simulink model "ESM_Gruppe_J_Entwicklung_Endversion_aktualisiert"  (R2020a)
settings: Solver=VariableStepAuto  StartTime=0  StopTime=Simulation  RelTol=1e-3
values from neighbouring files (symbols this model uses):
  c = [0;0]    [Testskript_Manoeverauswahl.m]
  ch = 100000    [Single_TestSkript_Hinterachse.m]    (also in Testskript_Hinterachse.m = 0)
  cv = 80000    [Single_Testskript_Vorderachse.m]    (also in Testskript_Vorderachse.m = (b-a).*rand(1,1) + a)
  Jzz = 1    [Single_Testskript_Karosserie.m]    (also in Testskript_Karosserie.m = (b-a).*rand(1,1) + a)
  lh = 1.3    [Single_TestSkript_Hinterachse.m]    (also in Testskript_Hinterachse.m = (b-a).*rand(1,1) + a; Single_Testskript_Karosserie.m; Testskript_Karosserie.m = (b-a).*rand(1,1) + a)
  lv = 1.3    [Single_Testskript_Karosserie.m]    (also in Testskript_Karosserie.m = (b-a).*rand(1,1) + a; Single_Testskript_Vorderachse.m = 1.5; Testskript_Vorderachse.m = (b-a).*rand(1,1) + a)
  m = 1500    [Single_Testskript_Karosserie.m]    (also in Testskript_Karosserie.m = (b-a).*rand(1,1) + a)

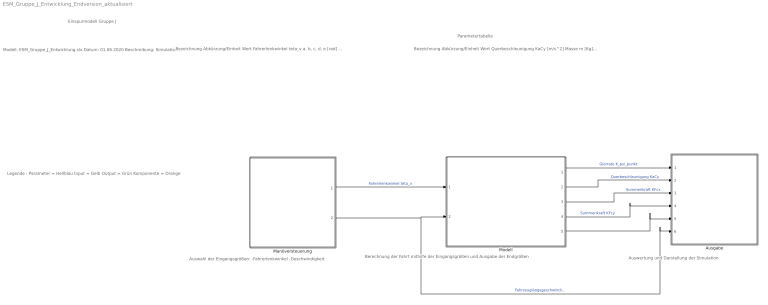
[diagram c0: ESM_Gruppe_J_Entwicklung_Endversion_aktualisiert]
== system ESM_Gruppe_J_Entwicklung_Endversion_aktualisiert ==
  note: Modell: ESM_Gruppe_J_Entwicklung.slx Datum: 01.06.2020 Beschreibung: Simulation der linearen Fahrdynamik Implementierung: Simulink 2019b (2019a) Autor: Alexander Gossen, Hermine Makou Bemerkung: Prototyp Letzte Änderung: 01.06.2020
  note: Bezeichnung Abkürzung/Einheit Wert Fahrerlenkwinkel teta_v a, b, c, d, e [rad] Fahrerlenkwinkel (hinten) teta_h 0 Fahrzeuglängsgeschwindigkeit KvCx a, b, c, d, e [m/s] Schwimmwinkel (vorne/hinten) beta, beta_v, beta_h [rad] Achschräglaufwinkel (vorne/hinten) Alpha_v, Alpha_h [rad] Seitenführungskraft (vorne/hinten) RFyv, RFyh [F] Gierrate K_psi_punkt
  note: Parametertabelle
  note: Einspurmodell Gruppe J
  note: Auswertung und Darstellung der Simulation
  note: Berechnung der Fahrt mithilfe der Eingangsgrößen und Ausgabe der Endgrößen
  note: Auswahl der Eingangsgrößen: -Fahrerlenkwinkel -Geschwindigkeit
  note: Legende : Parameter = Hellblau Input = Gelb Output = Grün Komponente = Orange
  note: Bezeichnung Abkürzung/Einheit Wert Querbeschleunigung KaCy [m/s^2] Masse m [Kg] 1550 Massenträgheit Jzz [Kg/m^2] 2800 Achsensteifigkeit (vorne/hinten) cv, ch [N/rad] 75.000 (vorne), 150.000 (hinten) Schwerpunktabstand (vorne/hinten) lv, lh [m] 1.3 (vorne), 2.6 (hinten) Radstand l
  Ausgabe : Subsystem
  Manöversteuerung : Subsystem
  Modell : Subsystem
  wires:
  Manöversteuerung/1(Fahrerlenkwinkel teta_v) -> Modell/1(Fahrerlenkwinkel teta_v)  "Fahrerlenkwinkel teta_v"
  Manöversteuerung/2(Fahrzeuglängsgeschwindigkeit KvCx) -> Modell/2(Fahrzeuglängsgeschwindigkeit KvCx), Ausgabe/6(Schwimmwinkel beta)  "Fahrzeuglängsgeschwindigkeit KvCx"
  Modell/1(Gierrate K_psi_punkt) -> Ausgabe/1(Gierrate K_psi_punkt)  "Gierrate K_psi_punkt"
  Modell/2(Querbeschleunigung KaCy) -> Ausgabe/2(Querbeschleunigung KaCy)  "Querbeschleunigung KaCy"
  Modell/3(Summenkraft KFcx) -> Ausgabe/3(Summenkraft KFcx)  "Summenkraft KFcx"
  Modell/4(Summenkraft KFcy) -> Ausgabe/4(Summenkraft KFcy)  "Summenkraft KFcy"
  Modell/5(Schwimmwinkel beta) -> Ausgabe/5(Fahrzeuglängsgeschwindigkeit KvCx)

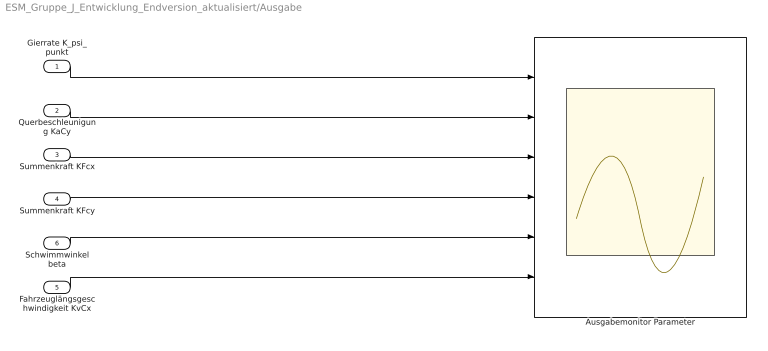
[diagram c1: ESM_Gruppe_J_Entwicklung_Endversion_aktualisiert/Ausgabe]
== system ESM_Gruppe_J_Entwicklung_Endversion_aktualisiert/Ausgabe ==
  Gierrate K_psi_punkt : Inport
  Querbeschleunigung KaCy : Inport  Port=2
  Summenkraft KFcx : Inport  Port=3
  Summenkraft KFcy : Inport  Port=4
  Fahrzeuglängsgeschwindigkeit KvCx : Inport  Port=5
  Schwimmwinkel beta : Inport  Port=6
  Ausgabemonitor Parameter : Scope  NumInputPorts=6
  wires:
  Gierrate K_psi_punkt/1 -> Ausgabemonitor Parameter/1
  Querbeschleunigung KaCy/1 -> Ausgabemonitor Parameter/2
  Summenkraft KFcx/1 -> Ausgabemonitor Parameter/3
  Summenkraft KFcy/1 -> Ausgabemonitor Parameter/4
  Schwimmwinkel beta/1 -> Ausgabemonitor Parameter/5
  Fahrzeuglängsgeschwindigkeit KvCx/1 -> Ausgabemonitor Parameter/6

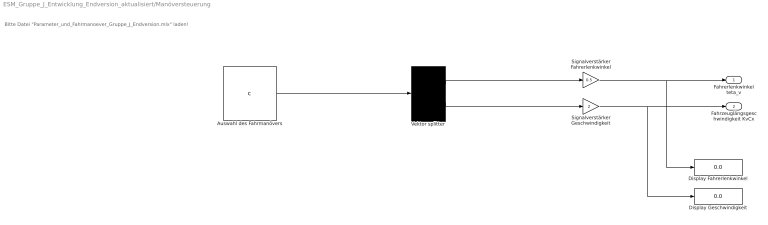
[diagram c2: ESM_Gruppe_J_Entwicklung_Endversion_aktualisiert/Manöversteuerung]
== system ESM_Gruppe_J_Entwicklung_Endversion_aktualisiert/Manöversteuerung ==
  note: Bitte Datei "Parameter_und_Fahrmanoever_Gruppe_J_Endversion.mlx" laden!
  Auswahl des Fahrmanövers : Constant  Value=c
  Display Fahrerlenkwinkel : Display
  Display Geschwindigkeit : Display
  Signalverstärker Fahrerlenkwinkel : Gain  Gain=0.5
  Signalverstärker Geschwindigkeit : Gain  Gain=2
  Vektor splitter : Demux  Outputs=2
  Fahrerlenkwinkel teta_v : Outport
  Fahrzeuglängsgeschwindigkeit KvCx : Outport  Port=2
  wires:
  Vektor splitter/1 -> Signalverstärker Fahrerlenkwinkel/1
  Vektor splitter/2 -> Signalverstärker Geschwindigkeit/1
  Signalverstärker Geschwindigkeit/1 -> Fahrzeuglängsgeschwindigkeit KvCx/1, Display Geschwindigkeit/1
  Signalverstärker Fahrerlenkwinkel/1 -> Fahrerlenkwinkel teta_v/1, Display Fahrerlenkwinkel/1
  Auswahl des Fahrmanövers/1 -> Vektor splitter/1

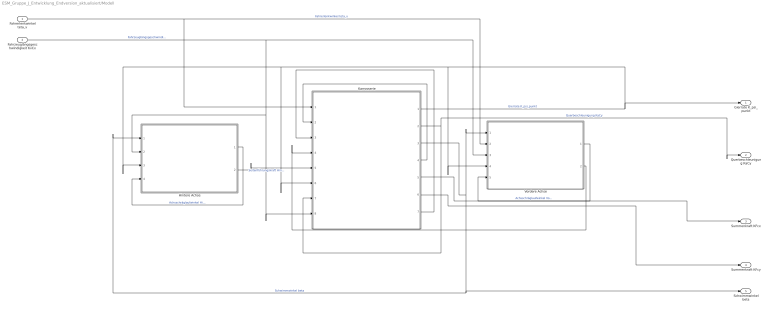
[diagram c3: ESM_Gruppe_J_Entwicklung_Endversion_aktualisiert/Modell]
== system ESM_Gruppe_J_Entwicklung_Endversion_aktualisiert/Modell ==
  Fahrerlenkwinkel teta_v : Inport
  Fahrzeuglängsgeschwindigkeit KvCx : Inport  Port=2
  Hintere Achse : Subsystem
  Karrosserie : Subsystem
  Vordere Achse : Subsystem
  Gierrate K_psi_punkt : Outport
  Querbeschleunigung KaCy : Outport  Port=2
  Summenkraft KFcx : Outport  Port=3
  Summenkraft KFcy : Outport  Port=4
  Schwimmwinkel beta : Outport  Port=5
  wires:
  Fahrerlenkwinkel teta_v/1 -> Vordere Achse/2(Fahrerlenkwinkel teta_v), Karrosserie/1(Fahrerlenkwinkel teta_v)  "Fahrerlenkwinkel teta_v"
  Fahrzeuglängsgeschwindigkeit KvCx/1 -> Vordere Achse/3(Geschwindigkeit KvCx), Karrosserie/8(Fahrzeuglängsgeschwindigkeit KvCx), Hintere Achse/2(Geschwindigkeit KvCx)  "Fahrzeuglängsgeschwindigkeit KvCx"
  Vordere Achse/1(Achsschräglaufwinkel vorderachse Alpha_v) -> Vordere Achse/5(Achsschräglaufwinkel vornerachse Alpha_v)  "Achsschräglaufwinkel Vorderachse Alpha_v"
  Hintere Achse/1(Achsschräglaufwinkel hinterachse alpha_v) -> Hintere Achse/4(Achsschräglaufwinkel hinterachse Alpha_h)  "Achsschräglaufwinkel Hinterachse Alpha_h"
  Vordere Achse/2(Seitenführungskraft vorderachse RFyv) -> Karrosserie/4(Seitenführungskraft vorderachse RFyv)
  Karrosserie/2(Querbeschleunigung kAcY) -> Karrosserie/7(Querbeschleunigung KaCy), Querbeschleunigung KaCy/1  "Querbeschleunigung KaCy"
  Karrosserie/1(Gierrate k_psi_punkt) -> Karrosserie/6(Gierrate K_psi_punkt), Hintere Achse/3(Gierrate K_psi_punkt), Vordere Achse/4(Gierrate K_psi_punkt), Gierrate K_psi_punkt/1  "Gierrate K_psi_punkt"
  Hintere Achse/2(Seitenführungskraft hinterachse RFyh) -> Karrosserie/5(Seitenführungskraft hintererachse RFyh)  "Seitenführungskraft Hinterachse RFyv"
  Karrosserie/6(Summenkraft KFcy) -> Summenkraft KFcy/1
  Karrosserie/5(Summenkraft KFcx) -> Summenkraft KFcx/1
  Karrosserie/4(Seitenführungskraft vorderachse KFyv) -> Karrosserie/2(Seitenführungskraft Vorderachse KFyv)
  Karrosserie/7(Seitenführungskraft hinterachse KFyh) -> Karrosserie/3(Seitenführungskraft Hinterachse KFyh)
  Karrosserie/3(Schwimmwinkel beta) -> Vordere Achse/1(Schwimmwinkel beta), Hintere Achse/1(Schwimmwinkel beta), Schwimmwinkel beta/1  "Schwimmwinkel beta"

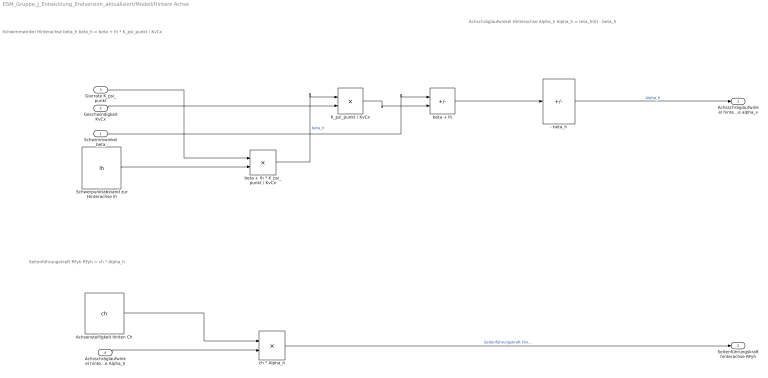
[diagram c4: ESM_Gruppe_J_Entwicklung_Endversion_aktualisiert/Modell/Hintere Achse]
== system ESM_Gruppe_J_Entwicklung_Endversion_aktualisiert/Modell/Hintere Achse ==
  note: Seitenführungskraft RFyh RFyh = ch * Alpha_h
  note: Schwimmwinkel Hinterachse beta_h beta_h = beta + Ih * K_psi_punkt / KvCx
  note: Achschräglaufwinkel Hinterachse Alpha_h Alpha_h = teta_h(0) - beta_h
  Schwimmwinkel beta : Inport
  Geschwindigkeit KvCx : Inport  Port=2
  Gierrate K_psi_punkt : Inport  Port=3
  Achsschräglaufwinkel hinterachse Alpha_h : Inport  Port=4
  - beta_h : Sum  Inputs=-
  Achsensteifigkeit hinten Ch : Constant  Value=ch
  K_psi_punkt / KvCx : Product  Inputs=*/
  Schwerpunktabstand zur Hinterachse lh : Constant  Value=lh
  beta + Ih : Sum  Inputs=+-
  beta + Ih * K_psi_punkt / KvCx : Product  Inputs=**
  ch * Alpha_h : Product
  Achsschräglaufwinkel hinterachse alpha_v : Outport
  Seitenführungskraft hinterachse RFyh : Outport  Port=2
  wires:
  - beta_h/1 -> Achsschräglaufwinkel hinterachse alpha_v/1  "Alpha_h"
  ch * Alpha_h/1 -> Seitenführungskraft hinterachse RFyh/1  "Seitenführungskraft Hinterachse RFyv"
  Achsensteifigkeit hinten Ch/1 -> ch * Alpha_h/1
  Achsschräglaufwinkel hinterachse Alpha_h/1 -> ch * Alpha_h/2
  beta + Ih * K_psi_punkt / KvCx/1 -> K_psi_punkt / KvCx/1  "beta_h"
  Geschwindigkeit KvCx/1 -> K_psi_punkt / KvCx/2
  beta + Ih/1 -> - beta_h/1
  Schwimmwinkel beta/1 -> beta + Ih/1
  K_psi_punkt / KvCx/1 -> beta + Ih/2
  Schwerpunktabstand zur Hinterachse lh/1 -> beta + Ih * K_psi_punkt / KvCx/2
  Gierrate K_psi_punkt/1 -> beta + Ih * K_psi_punkt / KvCx/1

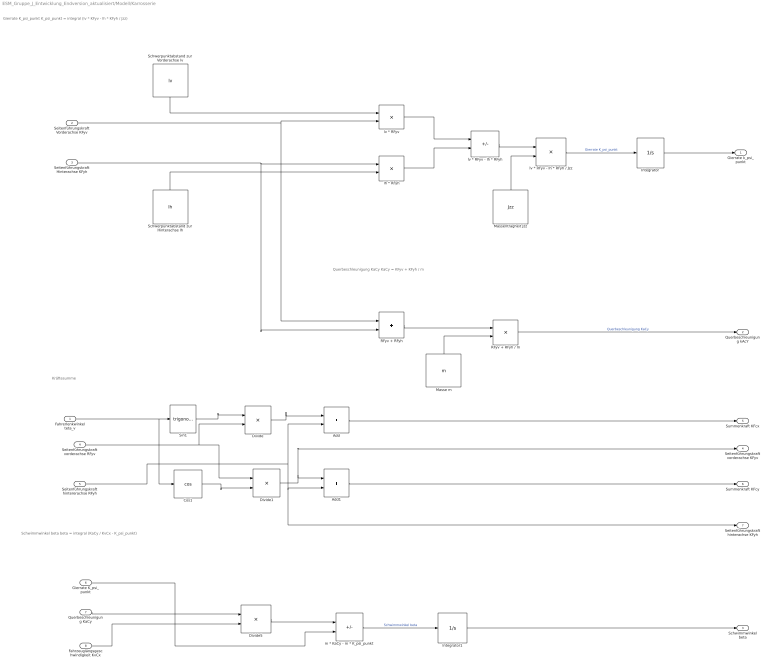
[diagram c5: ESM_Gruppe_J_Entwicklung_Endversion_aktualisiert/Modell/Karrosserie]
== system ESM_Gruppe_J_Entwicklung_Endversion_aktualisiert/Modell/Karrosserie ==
  note: Kräftesumme
  note: Gierrate K_psi_punkt K_psi_punkt = integral (lv * KFyv - lh * KFyh / Jzz)
  note: Querbeschleunigung KaCy KaCy = KFyv + KFyh / m
  note: Schwimmwinkel beta beta = integral (KaCy / KvCx - K_psi_punkt)
  Fahrerlenkwinkel teta_v : Inport
  Seitenführungskraft Vorderachse KFyv : Inport  Port=2
  Seitenführungskraft Hinterachse KFyh : Inport  Port=3
  Seitenführungskraft vorderachse RFyv : Inport  Port=4
  Seitenführungskraft hintererachse RFyh : Inport  Port=5
  Gierrate K_psi_punkt : Inport  Port=6
  Querbeschleunigung KaCy : Inport  Port=7
  Fahrzeuglängsgeschwindigkeit KvCx : Inport  Port=8
  Add : Sum
  Add1 : Sum
  Cos1 : Trigonometry  Operator=cos
  Divide : Product
  Divide1 : Product
  Divide5 : Product  Inputs=*/
  Integrator : Integrator
  Integrator1 : Integrator
  Masse m : Constant  Value=m
  Massenträgheit Jzz : Constant  Value=Jzz
  RFyv + RFyh : Sum
  RFyv + RFyh / m : Product  Inputs=*/
  Schwerpunktabstand zur Hinterachse lh : Constant  Value=lh
  Schwerpunktabstand zur Vorderachse lv : Constant  Value=lv
  Sin1 : Trigonometry
  lh * RFyh : Product
  lv * RFyv : Product
  lv * RFyv - lh * RFyh : Sum  Inputs=+-
  lv * RFyv - lh * RFyh / Jzz : Product  Inputs=*/
  m * KaCy - m * K_psi_punkt : Sum  Inputs=+-
  Gierrate k_psi_punkt : Outport
  Querbeschleunigung kAcY : Outport  Port=2
  Schwimmwinkel beta : Outport  Port=3
  Seitenführungskraft vorderachse KFyv : Outport  Port=4
  Summenkraft KFcx : Outport  Port=5
  Summenkraft KFcy : Outport  Port=6
  Seitenführungskraft hinterachse KFyh : Outport  Port=7
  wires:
  RFyv + RFyh / m/1 -> Querbeschleunigung kAcY/1  "Querbeschleunigung KaCy"
  m * KaCy - m * K_psi_punkt/1 -> Integrator1/1  "Schwimmwinkel beta"
  lv * RFyv - lh * RFyh/1 -> lv * RFyv - lh * RFyh / Jzz/1
  lv * RFyv/1 -> lv * RFyv - lh * RFyh/1
  Massenträgheit Jzz/1 -> lv * RFyv - lh * RFyh / Jzz/2
  lh * RFyh/1 -> lv * RFyv - lh * RFyh/2
  Schwerpunktabstand zur Vorderachse lv/1 -> lv * RFyv/1
  Schwerpunktabstand zur Hinterachse lh/1 -> lh * RFyh/2
  Masse m/1 -> RFyv + RFyh / m/2
  RFyv + RFyh/1 -> RFyv + RFyh / m/1
  Fahrerlenkwinkel teta_v/1 -> Cos1/1, Sin1/1
  Sin1/1 -> Divide/1
  Seitenführungskraft vorderachse RFyv/1 -> Divide1/1, Divide/2
  Divide/1 -> Add/1
  Seitenführungskraft hintererachse RFyh/1 -> Add/2, Seitenführungskraft hinterachse KFyh/1, Add1/2
  Add/1 -> Summenkraft KFcx/1
  Divide1/1 -> Seitenführungskraft vorderachse KFyv/1, Add1/1
  Add1/1 -> Summenkraft KFcy/1
  Seitenführungskraft Vorderachse KFyv/1 -> RFyv + RFyh/1, lv * RFyv/2
  Seitenführungskraft Hinterachse KFyh/1 -> RFyv + RFyh/2, lh * RFyh/1
  Querbeschleunigung KaCy/1 -> Divide5/1
  Fahrzeuglängsgeschwindigkeit KvCx/1 -> Divide5/2
  Divide5/1 -> m * KaCy - m * K_psi_punkt/1
  Gierrate K_psi_punkt/1 -> m * KaCy - m * K_psi_punkt/2
  Integrator1/1 -> Schwimmwinkel beta/1
  lv * RFyv - lh * RFyh / Jzz/1 -> Integrator/1  "Gierrate K_psi_punkt"
  Integrator/1 -> Gierrate k_psi_punkt/1
  Cos1/1 -> Divide1/2

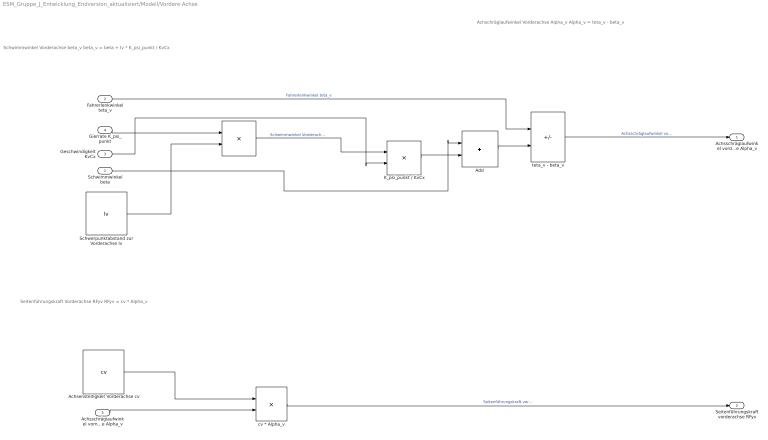
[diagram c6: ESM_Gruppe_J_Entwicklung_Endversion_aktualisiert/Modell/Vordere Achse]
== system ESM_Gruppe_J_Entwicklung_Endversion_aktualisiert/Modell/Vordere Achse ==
  note: Seitenführungskraft Vorderachse RFyv RFyv = cv * Alpha_v
  note: Schwimmwinkel Vorderachse beta_v beta_v = beta + Iv * K_psi_punkt / KvCx
  note: Achschräglaufwinkel Vorderachse Alpha_v Alpha_v = teta_v - beta_v
  Schwimmwinkel beta : Inport
  Fahrerlenkwinkel teta_v : Inport  Port=2
  Geschwindigkeit KvCx : Inport  Port=3
  Gierrate K_psi_punkt : Inport  Port=4
  Achsschräglaufwinkel vornerachse Alpha_v : Inport  Port=5
  " " : Product  Inputs=**
  Achsensteifigkeit Vorderachse cv : Constant  Value=cv
  Add : Sum
  K_psi_punkt / KvCx : Product  Inputs=*/
  Schwerpunktabstand zur Vorderachse lv : Constant  Value=lv
  cv * Alpha_v : Product
  teta_v - beta_v : Sum  Inputs=+-
  Achsschräglaufwinkel vorderachse Alpha_v : Outport
  Seitenführungskraft vorderachse RFyv : Outport  Port=2
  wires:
  teta_v - beta_v/1 -> Achsschräglaufwinkel vorderachse Alpha_v/1  "Achsschräglaufwinkel vorderachse Alpha_v"
  cv * Alpha_v/1 -> Seitenführungskraft vorderachse RFyv/1  "Seitenführungskraft vorderachse RFyv"
  Achsensteifigkeit Vorderachse cv/1 -> cv * Alpha_v/1
  Achsschräglaufwinkel vornerachse Alpha_v/1 -> cv * Alpha_v/2
  " "/1 -> K_psi_punkt / KvCx/1  "Schwimmwinkel Vorderachse beta_v"
  Geschwindigkeit KvCx/1 -> K_psi_punkt / KvCx/2
  Fahrerlenkwinkel teta_v/1 -> teta_v - beta_v/1  "Fahrerlenkwinkel teta_v"
  Schwimmwinkel beta/1 -> Add/1
  K_psi_punkt / KvCx/1 -> Add/2
  Add/1 -> teta_v - beta_v/2
  Gierrate K_psi_punkt/1 -> " "/1
  Schwerpunktabstand zur Vorderachse lv/1 -> " "/2
